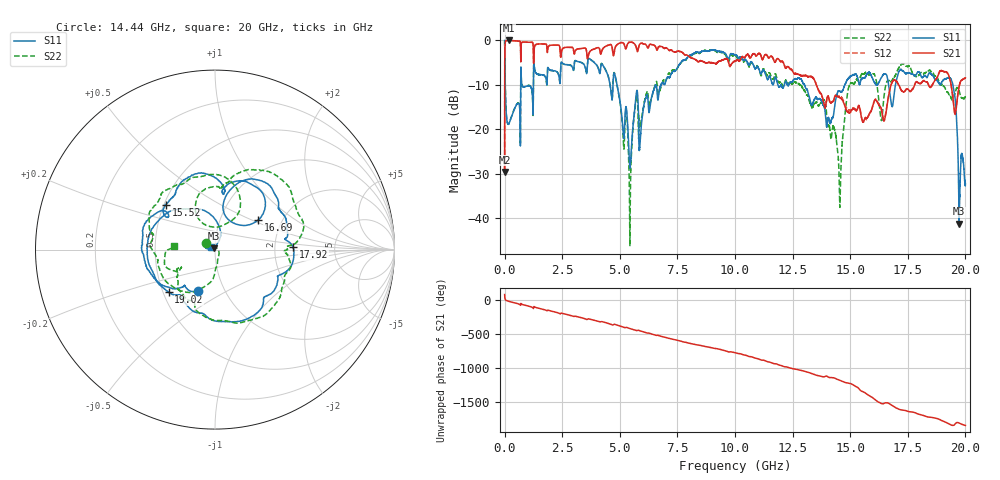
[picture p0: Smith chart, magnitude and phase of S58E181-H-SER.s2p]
!{S58E181}
!Johanson Technology Inc.
!www.johansontechnology.com
!Test Board Conditions:
!Substrate Type  RO4350B
!Substrate Thickness  60 mil
!Substrate Dk  3.66
!TL Type: GCPW
!TL Trace Width  115 mil
!TL Gap  52 mil
!Electrode orientation  Horizontal
!DUT TOPOLOGY	SERIES
!Mounting Pad LxW  55x428 mil
! Created Wed Apr 14 11:24:34 2021
# mhz S ma R 50
! 2 Port Network Data from SP1.SP block
! freq  magS11  angS11  magS21  angS21  magS12  angS12  magS22  angS22
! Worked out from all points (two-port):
!   20001 points, 300 kHz to 20 GHz, reference 50 ohm
!   highest |S21| = -0.06 dB at 202.3 MHz (marker M1); lowest = -29.6 dB at 300 kHz (marker M2)
!   |S21| within 3 dB of the highest: 1.273 GHz to 2.419 GHz (1.146 GHz wide, 62.1 % of centre); 4.745 GHz to 7.768 GHz (3.023 GHz wide, 48.3 % of centre)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
!   lowest |S11| = -41.3 dB at 19.73 GHz (marker M3), VSWR 1.02, Z = 49.5 + j0.727 ohm
!   |S11| at or under -10 dB: 27.75 MHz to 699.8 MHz (672.1 MHz wide, 185 % of centre); 4.879 GHz to 6.794 GHz (1.914 GHz wide, 32.8 % of centre); 13.01 GHz to 14.77 GHz (1.763 GHz wide, 12.7 % of centre)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
!   |S22| runs from -46.3 to -0.1 dB; largest |S21 - S12| = 0.013
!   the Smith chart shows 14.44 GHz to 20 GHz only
!   S11 on the Smith chart (normalised r, x): 14.44 GHz: 0.74, -0.37; 15.52 GHz: 0.51, +0.30; 16.69 GHz: 1.51, +0.54; 17.92 GHz: 2.54, +0.08; 19.02 GHz: 0.53, -0.29; 20 GHz: 0.96, +0.03
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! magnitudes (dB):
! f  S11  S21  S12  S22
! 300 kHz  -0.1  -29.6  -29.6  -0.1
! 102.3 MHz  -18.1  -0.1  -0.1  -18.1
! 202.3 MHz  -18.5  -0.1  -0.1  -18.5
! 1.353 GHz  -7.3  -1.0  -1.0  -7.3
! 3.334 GHz  -5.0  -1.9  -1.9  -5.0
! 4.815 GHz  -8.4  -1.5  -1.5  -8.4
! 5.448 GHz  -28.7  -0.5  -0.4  -38.6
! 5.685 GHz  -13.5  -1.2  -1.2  -13.9
! 5.912 GHz  -20.7  -0.7  -0.7  -18.7
! 6.667 GHz  -13.2  -1.6  -1.6  -12.0
! 10 GHz  -3.4  -4.7  -4.7  -3.6
! 13.33 GHz  -14.5  -8.3  -8.2  -15.2
! 14.44 GHz  -12.0  -12.6  -12.6  -24.0
! 15.52 GHz  -8.6  -18.0  -17.8  -7.5
! 16.34 GHz  -8.5  -15.4  -15.2  -17.9
! 16.67 GHz  -10.1  -12.5  -12.4  -9.1
! 16.69 GHz  -10.8  -12.0  -11.9  -9.1
! 17.92 GHz  -7.2  -9.5  -9.4  -8.1
! 19.02 GHz  -9.1  -7.0  -7.0  -10.1
! 19.48 GHz  -10.7  -14.0  -13.9  -12.9
! 19.73 GHz  -41.3  -10.4  -10.4  -11.4
! 20 GHz  -32.3  -8.5  -8.4  -12.8
